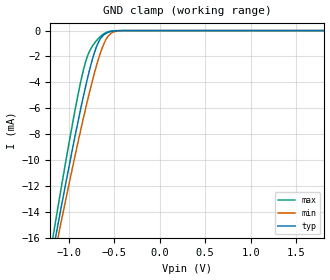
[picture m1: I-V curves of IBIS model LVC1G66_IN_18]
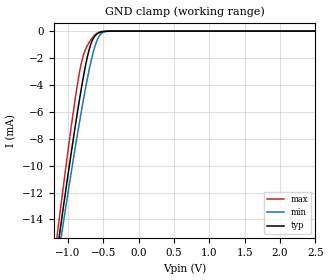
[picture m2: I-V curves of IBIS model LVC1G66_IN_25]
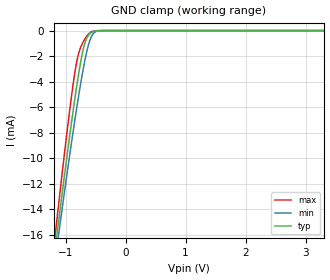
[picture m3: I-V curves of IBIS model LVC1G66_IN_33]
| TEXAS INSTRUMENTS INCORPORATED
| Standard Linear and Logic Group
| IBIS Model of SN74LVC1G66
| SINGLE BILATERAL ANALOG SWITCH
| This file contains package information for the following:
|  SOT 5-pin (DBV) package as [Component] LVC1G66_DBV
|  SOT 5-pin (DCK) package as [Component] LVC1G66_DCK
|  SOT 5-pin (DRL) package as [Component] LVC1G66_DRL
|  NanoStar WCSP 5-pin (YEA) package as [Component] LVC1G66_YEA
|  NanoFree WCSP 5-pin (YZA) package as [Component] LVC1G66_YZA
|  NanoStar WCSP 5-pin (YEP) package as [Component] LVC1G66_YEP
|  NanoFree WCSP 5-pin (YZP) package as [Component] LVC1G66_YZP
| This device can be powered at the following Vccs:
|  1.8 volt Vcc
|  2.5 volt Vcc
|  3.3 volt Vcc
|  5 volt Vcc
| This file provides unique models under the [Model Selector] for each Vcc.
| For operation at a specific Vcc, select the appropriate model after each
| [Model Selector] keyword.
[IBIS Ver]   3.2
[Comment char]  |_char
[File Name]   sn74lvc1g66.ibs
[File Rev]   1.3 | x_die
[Date]   May 15, 2004
[Source]   Data created from TI-SPICE simulations at TI-SLL.
[Notes]   The following is an IBIS list for the SN74LVC1G66.
   Please contact sllibis@ti.com with questions and
   comments concerning SLL IBIS models.
   - FILE REV HISTORY
   - 1.2 YEP and YZP packages added on 05/15/04
   - 1.3 DRL package added on 1/16/2008
   - As there is no power clamp diode in the Input Models,
   we removed the power clamp table data from those
   Models.
   - C_comp values are taken at a different test condition than
   the Ci and Cio in data sheet.
[Disclaimer] Property of Texas Instruments Incorporated.  Unauthorized
   reproduction and/or distribution is strictly prohibited.
   This product is protected under copyright law.
   Created  2002, (C) Copyright  2002, Texas Instruments
   Incorporated, All Rights Reserved
   UNLESS THERE IS A SIGNED, WRITTEN AGREEMENT TO THE
   CONTRARY, TEXAS INSTRUMENTS (TI) IS PROVIDING THE IBIS
   MODELS  AND WITHOUT ANY WARRANTY, EXPRESSED OR
   IMPLIED.  TI assumes no liability for:
   1) the accuracy of the IBIS models provided to your
   company;
   2) the proper functioning of these IBIS Models in your
   design or for any resulting applications; or
   3) infringement of patents, copyrights or intellectual
   property rights resulting from your use of these IBIS
   models.
   TI provides IBIS Models as a service to our customers.
   You and your company shall not distribute, sell or give
   these models to anyone else without prior written
   permission from TI.
   TI reserves the right to make changes to our products or
   to discontinue any semiconductor product or service
   without notice, and advises our customers to obtain the
   latest version of relevant information to verify, before
   placing orders, that the information being relied on is
   current.
   Please be aware that your receipt and use of the IBIS
   information provided shall serve as acceptance of these
   terms and conditions.  If you do not accept these terms,
   you should return or destroy the IBIS models and any
   other accompanying information immediately.
| Component LVC1G66_DBV 5-pin SOT
[Component]   LVC1G66_DBV
[Manufacturer]  Texas Instruments, Inc.
[Package]
|   typ   min   max
R_pkg   2.500e-02   2.100e-02   2.900e-02
L_pkg   1.529e-09   1.312e-09   1.906e-09
C_pkg   1.560e-13   1.100e-13   2.400e-13
[Pin]   signal_name   model_name   R_pin   L_pin   C_pin
1   A   LVC1G66_IO   2.100e-02   1.511e-09   1.440e-13
2   B   LVC1G66_IO   2.300e-02   1.312e-09   1.380e-13
3   GND   GND   2.900e-02   1.906e-09   2.400e-13
4   C   LVC1G66_IN   2.600e-02   1.541e-09   1.500e-13
5   VCC   POWER   2.500e-02   1.374e-09   1.100e-13
| Component LVC1G66_DCK 5-pin SOT
[Component]   LVC1G66_DCK
[Manufacturer]  Texas Instruments, Inc.
[Package]
|   typ   min   max
R_pkg   2.000e-02   1.700e-02   2.500e-02
L_pkg   9.980e-10   8.810e-10   1.069e-09
C_pkg   1.460e-13   1.180e-13   2.050e-13
[Pin]   signal_name   model_name   R_pin   L_pin   C_pin
1   A   LVC1G66_IO   1.900e-02   1.069e-09   1.620e-13
2   B   LVC1G66_IO   1.800e-02   8.810e-10   1.210e-13
3   GND   GND   1.700e-02   1.031e-09   2.050e-13
4   C   LVC1G66_IN   2.000e-02   9.600e-10   1.240e-13
5   VCC   POWER   2.500e-02   1.049e-09   1.180e-13
| Component LVC1G66_DRL 5-PIN SOT
[Component]   LVC1G66_DRL
[Manufacturer]   Texas Instruments, Inc.
[Package]
|   typ   min   max
R_pkg   3.200e-02   2.800e-02   3.500e-02
L_pkg   9.160e-10   7.230e-10   1.135e-09
C_pkg   2.210e-13   1.030e-13   3.740e-13
[Pin]   signal_name   model_name   R_pin   L_pin   C_pin
1   A   LVC1G66_IO   3.400e-02   7.230e-10   1.030e-13
2   B   LVC1G66_IO   2.800e-02   8.930e-10   2.370e-13
3   GND   GND   2.900e-02   1.072e-09   3.740e-13
4   C   LVC1G66_IN   3.500e-02   7.600e-10   1.130e-13
5   VCC   POWER   3.300e-02   1.135e-09   2.800e-13
| Component LVC1G66_YEA 5-pin NanoStar WCSP
[Component]   LVC1G66_YEA
[Manufacturer]   Texas Instruments, Inc.
[Package]
|   typ   min   max
R_pkg   0.001   0.001   0.001
L_pkg   0.021nH   0.021nH   0.021nH
C_pkg   0.046pF   0.045pF   0.047pF
[Pin]   signal_name   model_name   R_pin   L_pin   C_pin
1   A   LVC1G66_IO   0.001   0.021nH   0.046pF
2   B   LVC1G66_IO   0.001   0.021nH   0.047pF
3   GND   GND   0.001   0.021nH   0.046pF
4   C   LVC1G66_IN   0.001   0.021nH   0.045pF
5   VCC   POWER   0.001   0.021nH   0.045pF
| Component LVC1G66_YZA 5-pin NanoFree WCSP
[Component]   LVC1G66_YZA
[Manufacturer]   Texas Instruments, Inc.
[Package]
|   typ   min   max
R_pkg   0.001   0.001   0.001
L_pkg   0.021nH   0.021nH   0.021nH
C_pkg   0.046pF   0.045pF   0.047pF
[Pin]   signal_name   model_name   R_pin   L_pin   C_pin
1   A   LVC1G66_IO   0.001   0.021nH   0.046pF
2   B   LVC1G66_IO   0.001   0.021nH   0.047pF
3   GND   GND   0.001   0.021nH   0.046pF
4   C   LVC1G66_IN   0.001   0.021nH   0.045pF
5   VCC   POWER   0.001   0.021nH   0.045pF
| Component LVC1G66_YEP 5-pin NanoStar WCSP
[Component]   LVC1G66_YEP
[Manufacturer]   Texas Instruments, Inc.
[Package]
|   typ   min   max
R_pkg   0.001   0.001   0.001
L_pkg   0.021nH   0.021nH   0.021nH
C_pkg   0.046pF   0.045pF   0.047pF
[Pin]   signal_name   model_name   R_pin   L_pin   C_pin
1   A   LVC1G66_IO   0.001   0.021nH   0.046pF
2   B   LVC1G66_IO   0.001   0.021nH   0.047pF
3   GND   GND   0.001   0.021nH   0.046pF
4   C   LVC1G66_IN   0.001   0.021nH   0.045pF
5   VCC   POWER   0.001   0.021nH   0.045pF
| Component LVC1G66_YZP 5-pin NanoFree WCSP
[Component]   LVC1G66_YZP
[Manufacturer]   Texas Instruments, Inc.
[Package]
|   typ   min   max
R_pkg   0.001   0.001   0.001
L_pkg   0.021nH   0.021nH   0.021nH
C_pkg   0.046pF   0.045pF   0.047pF
[Pin]   signal_name   model_name   R_pin   L_pin   C_pin
1   A   LVC1G66_IO   0.001   0.021nH   0.046pF
2   B   LVC1G66_IO   0.001   0.021nH   0.047pF
3   GND   GND   0.001   0.021nH   0.046pF
4   C   LVC1G66_IN   0.001   0.021nH   0.045pF
5   VCC   POWER   0.001   0.021nH   0.045pF
[Series Switch Groups]
| Function Group States
On  1 /   | A->B C HIGH
[Series Pin Mapping]   pin_2   model_name   function_table_group
1   2   LVC1G66_IO_18_S   1
| 1   2   LVC1G66_IO_25_S   1
| 1   2   LVC1G66_IO_33_S   1
| 1   2   LVC1G66_IO_50_S   1
| Model LVC1G66_IN
[Model Selector]   LVC1G66_IN
LVC1G66_IN_18   1.8 volt Vcc
LVC1G66_IN_25   2.5 volt Vcc
LVC1G66_IN_33   3.3 volt Vcc
LVC1G66_IN_50   5 volt Vcc
| Model LVC1G66_IO
[Model Selector]   LVC1G66_IO
LVC1G66_IO_18   1.8 volt Vcc
LVC1G66_IO_25   2.5 volt Vcc
LVC1G66_IO_33   3.3 volt Vcc
LVC1G66_IO_50   5 volt Vcc
| Model LVC1G66_IO
[Model Selector]   LVC1G66_IO_S
LVC1G66_IO_18_S   1.8 volt Vcc
LVC1G66_IO_25_S   2.5 volt Vcc
LVC1G66_IO_33_S   3.3 volt Vcc
LVC1G66_IO_50_S   5 volt Vcc
[Model]   LVC1G66_IO_18_S
Model_type  Series_switch
| variable   typ   min   max
C_comp   0   0   0
[Temperature Range]   40   100   -40
| Ambient temperature   25   85   -40
[Voltage range]   1.8   1.65   1.95
[On]
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[Off]
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[Model]   LVC1G66_IO_25_S
Model_type  Series_switch
| variable   typ   min   max
C_comp   0   0   0
[Temperature Range]   40   100   -40
| Ambient temperature   25   85   -40
[Voltage range]   2.5   2.3   2.7
[On]
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[Off]
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[Model]   LVC1G66_IO_33_S
Model_type  Series_switch
| variable   typ   min   max
C_comp   0   0   0
[Temperature Range]   40   100   -40
| Ambient temperature   25   85   -40
[Voltage range]   3.3   3   3.6
[On]
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[Off]
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[Model]   LVC1G66_IO_50_S
Model_type  Series_switch
| variable   typ   min   max
C_comp   0   0   0
[Temperature Range]   40   100   -40
| Ambient temperature   25   85   -40
[Voltage range]   5   4.5   5.5
[On]
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[Off]
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| Models and submodels in the file (12): LVC1G66_IN_18 (Input), LVC1G66_IN_25 (Input), LVC1G66_IN_33 (Input), LVC1G66_IN_50 (Input), LVC1G66_IO_18_S (Series_switch), LVC1G66_IO_18 (Terminator), LVC1G66_IO_25_S (Series_switch), LVC1G66_IO_25 (Terminator), LVC1G66_IO_33_S (Series_switch), LVC1G66_IO_33 (Terminator), LVC1G66_IO_50_S (Series_switch), LVC1G66_IO_50 (Terminator)
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[Model]   LVC1G66_IN_18
Model_type  Input
Vinl=0.5775
Vinh=1.2675
| variable   typ   min   max
C_comp   2.97pF   2.67pF   3.28pF
[Temperature Range]   40   100   -40
| Ambient temperature   25   85   -40
[Voltage range]   1.8   1.65   1.95
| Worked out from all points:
|   GND clamp passes 1 mA (typ) near -0.68 V on its own axis
[GND Clamp]
| LVC1G66_IN_18
|   Voltage   I(typ)   I(min)   I(max)
-5.5V     -200.6mA   -187.3mA   -217mA
-1.16V    -16.65mA   -17.52mA   -15.49mA
-1.125V   -15.33mA   -16.31mA   -14.02mA
-1.09V    -14.01mA   -15.1mA    -12.56mA
-930mV    -8.212mA   -9.724mA   -6.206mA
-825mV    -4.706mA   -6.402mA   -2.73mA
-775mV    -3.204mA   -4.916mA   -1.679mA
-700mV    -1.375mA   -2.878mA   -836.9uA
-605mV    -289.7uA   -916uA     -219.5uA
-530mV    -68.42uA   -194.4uA   -38.21uA
-410mV    -3.575uA   -8.117uA   -762.4nA
1.8V      32.58pA    92.8pA     21.64pA
[Model]   LVC1G66_IN_25
Model_type  Input
Vinl=0.69
Vinh=1.89
| variable   typ   min   max
C_comp   2.92pF   2.63pF   3.27pF
[Temperature Range]   40   100   -40
| Ambient temperature   25   85   -40
[Voltage range]   2.5   2.3   2.7
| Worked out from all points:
|   GND clamp passes 1 mA (typ) near -0.68 V on its own axis
[GND Clamp]
| LVC1G66_IN_25
|   Voltage   I(typ)   I(min)   I(max)
-5.5V     -200.6mA   -187.3mA   -217mA
-1.16V    -16.65mA   -17.52mA   -15.49mA
-1.125V   -15.33mA   -16.31mA   -14.02mA
-1.095V   -14.2mA    -15.27mA   -12.77mA
-1.065V   -13.08mA   -14.24mA   -11.53mA
-915mV    -7.692mA   -9.237mA   -5.653mA
-805mV    -4.087mA   -5.798mA   -2.243mA
-725mV    -1.906mA   -3.525mA   -1.069mA
-670mV    -874.2uA   -2.161mA   -596.2uA
-595mV    -242.6uA   -773uA     -180.7uA
-520mV    -55.05uA   -151.8uA   -28.9uA
2.5V      44.7pA     113pA      30.06pA
[Model]   LVC1G66_IN_33
Model_type  Input
Vinl=0.9
Vinh=2.52
| variable   typ   min   max
C_comp   2.88pF   2.57pF   3.27pF
[Temperature Range]   40   100   -40
| Ambient temperature   25   85   -40
[Voltage range]   3.3   3   3.6
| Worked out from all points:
|   GND clamp passes 1 mA (typ) near -0.68 V on its own axis
[GND Clamp]
| LVC1G66_IN_33
|   Voltage   I(typ)   I(min)   I(max)
-5.5V     -200.6mA   -187.3mA   -217mA
-1.195V   -17.98mA   -18.75mA   -16.97mA
-1.16V    -16.65mA   -17.52mA   -15.49mA
-1.125V   -15.33mA   -16.31mA   -14.02mA
-1.09V    -14.01mA   -15.1mA    -12.56mA
-925mV    -8.038mA   -9.561mA   -6.02mA
-805mV    -4.087mA   -5.798mA   -2.243mA
-730mV    -2.024mA   -3.658mA   -1.119mA
-665mV    -806.4uA   -2.049mA   -559.9uA
-585mV    -202.6uA   -644.7uA   -146.9uA
-510mV    -44.01uA   -117.8uA   -21.65uA
3.3V      59.38pA    137.5pA    39.69pA
